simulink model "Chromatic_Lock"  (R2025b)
settings: Solver=FixedStepDiscrete  StartTime=0.0  StopTime=inf  FixedStep=0.01  RelTol=1e-3  EnableMultiTasking=on
libraries: arduinolib x3
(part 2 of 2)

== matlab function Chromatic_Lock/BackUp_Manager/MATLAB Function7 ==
function [RGB, L1, L2, L3, L4, Tone_Event] = ...
    Game_Manager(R_idx, G_idx, B_idx, Match_Btn, Select_Btn, Difficulty_Input, Reset_Btn)
%#codegen

%% ================= DATA TYPES =================
R_idx = uint8(R_idx);
G_idx = uint8(G_idx);
B_idx = uint8(B_idx);
Difficulty_Input = uint8(Difficulty_Input);

% Clamp encoder indices to valid palette range
R_idx = max(uint8(1), min(uint8(6), R_idx));
G_idx = max(uint8(1), min(uint8(6), G_idx));
B_idx = max(uint8(1), min(uint8(6), B_idx));

% Clamp difficulty
Difficulty_Input = max(uint8(1), min(uint8(3), Difficulty_Input));

%% ============ PERSISTENT VARIABLES ============
persistent state puzzle_count puzzle_limit ...
    R_tgt G_tgt B_tgt ...
    R_hints G_hints B_hints

if isempty(state)
    state = uint8(0);  % welcome screen        % 0=Select Difficulty, 1=Play, 2=Complete
    puzzle_count = uint8(1);
    puzzle_limit = uint8(0);

    % --- Targets as numeric arrays (6 puzzles) ---
    R_tgt = zeros(6,1,'uint8');
    G_tgt = zeros(6,1,'uint8');
    B_tgt = zeros(6,1,'uint8');

    % --- Hints as cell arrays (6 puzzles x 3 difficulty levels) ---
    R_hints = cell(6,3);
    G_hints = cell(6,3);
    B_hints = cell(6,3);

    % ==================== PUZZLES ====================
    % PUZZLE 1
    R_tgt(1) = 2; R_hints{1,1} = 'Rot: Tomatenrot      '; R_hints{1,2} = 'Rot: Ziegelrot       '; R_hints{1,3} = 'Rot: Scharlach       ';
    G_tgt(1) = 1; G_hints{1,1} = 'Gruen: Apfelgruen    '; G_hints{1,2} = 'Gruen: Fruehlingsgruen'; G_hints{1,3} = 'Gruen: Moosgruen      ';
    B_tgt(1) = 3; B_hints{1,1} = 'Blau: Azurblau       '; B_hints{1,2} = 'Blau: EU-Blau        '; B_hints{1,3} = 'Blau: Koenigsblau     ';

    % PUZZLE 2
    R_tgt(2) = 4; R_hints{2,1} = 'Rot: Kirschrot       '; R_hints{2,2} = 'Rot: Rubinrot        '; R_hints{2,3} = 'Rot: Purpur          ';
    G_tgt(2) = 3; G_hints{2,1} = 'Gruen: Hoffnungsgruen'; G_hints{2,2} = 'Gruen: Smaragd       '; G_hints{2,3} = 'Gruen: Tannengruen    ';
    B_tgt(2) = 5; B_hints{2,1} = 'Blau: Marineblau     '; B_hints{2,2} = 'Blau: Tiefsee        '; B_hints{2,3} = 'Blau: Mitternacht    ';

    % PUZZLE 3
    R_tgt(3) = 6; R_hints{3,1} = 'Rot: Feuerrot        '; R_hints{3,2} = 'Rot: Glutrot         '; R_hints{3,3} = 'Rot: Vulkanrot       ';
    G_tgt(3) = 1; G_hints{3,1} = 'Gruen: Apfelgruen    '; G_hints{3,2} = 'Gruen: Limette       '; G_hints{3,3} = 'Gruen: Farn          ';
    B_tgt(3) = 3; B_hints{3,1} = 'Blau: Heraldik       '; B_hints{3,2} = 'Blau: Stahlblau      '; B_hints{3,3} = 'Blau: Polarblau      ';

    % PUZZLE 4
    R_tgt(4) = 3; R_hints{4,1} = 'Rot: Ziegelrot       '; R_hints{4,2} = 'Rot: Terrakotta      '; R_hints{4,3} = 'Rot: Ockerrot        ';
    G_tgt(4) = 4; G_hints{4,1} = 'Gruen: Limettengruen '; G_hints{4,2} = 'Gruen: Chartreuse    '; G_hints{4,3} = 'Gruen: Neon          ';
    B_tgt(4) = 2; B_hints{4,1} = 'Blau: Mittelmeer     '; B_hints{4,2} = 'Blau: Kuestenblau    '; B_hints{4,3} = 'Blau: Horizont       ';

    % PUZZLE 5
    R_tgt(5) = 5; R_hints{5,1} = 'Rot: Rosenrot        '; R_hints{5,2} = 'Rot: Altrosa         '; R_hints{5,3} = 'Rot: Pastellrot      ';
    G_tgt(5) = 6; G_hints{5,1} = 'Gruen: Dschungelgruen'; G_hints{5,2} = 'Gruen: Tropengruen   '; G_hints{5,3} = 'Gruen: Mangroven     ';
    B_tgt(5) = 1; B_hints{5,1} = 'Blau: Eisblau        '; B_hints{5,2} = 'Blau: EU-Blau        '; B_hints{5,3} = 'Blau: Stahlblau      ';

    % PUZZLE 6
    R_tgt(6) = 1; R_hints{6,1} = 'Rot: Tomatenrot      '; R_hints{6,2} = 'Rot: Bordeaux        '; R_hints{6,3} = 'Rot: Burgunder       ';
    G_tgt(6) = 2; G_hints{6,1} = 'Gruen: Irischgruen   '; G_hints{6,2} = 'Gruen: Moosgruen     '; G_hints{6,3} = 'Gruen: Waldgruen     ';
    B_tgt(6) = 5; B_hints{6,1} = 'Blau: Marineblau     '; B_hints{6,2} = 'Blau: Tiefsee        '; B_hints{6,3} = 'Blau: Nachtblau      ';
end

%% ================= RESET ======================
if Reset_Btn
    state = uint8(0);   % welcome screen
    puzzle_count = uint8(1);
    puzzle_limit = uint8(0);
end

%% ================= DEFAULT OUTPUTS ============
RGB = [0.2 0.2 0.2];
Tone_Event = uint8(0);

L1 = uint8('                    ');
L2 = uint8('                    ');
L3 = uint8('                    ');
L4 = uint8('                    ');

palette = [1.0 0.8 0.6 0.4 0.2 0.1];

%% ================= FSM ========================
switch state

    % ========== STATE 0: WELCOME SCREEN ==========
    case 0
        L1 = uint8('   Chromatic Lock   ');
        L2 = uint8('       Bereit       ');
        L3 = uint8('                    ');
        L4 = uint8('Druecke zum Starten ');

        if Select_Btn
            state = uint8(1);
        end

    % ========== STATE 1: SELECT DIFFICULTY ==========
    case 1
        L1 = uint8('-- SCHWIERIGKEIT -- ');

        % --- Visual feedback for selection ---
        if Difficulty_Input == 1
            L2 = uint8('> 1 LEICHT          ');
            L3 = uint8('  2 MITTEL          ');
            L4 = uint8('  3 SCHWER          ');
        elseif Difficulty_Input == 2
            L2 = uint8('  1 LEICHT          ');
            L3 = uint8('> 2 MITTEL          ');
            L4 = uint8('  3 SCHWER          ');
        elseif Difficulty_Input == 3
            L2 = uint8('  1 LEICHT          ');
            L3 = uint8('  2 MITTEL          ');
            L4 = uint8('> 3 SCHWER          ');
        end

        if Select_Btn
            if Difficulty_Input == 1
                puzzle_limit = uint8(3);
            elseif Difficulty_Input == 2
                puzzle_limit = uint8(4);
            elseif Difficulty_Input == 3
                puzzle_limit = uint8(6);
            else
                puzzle_limit = uint8(0);
            end

            if puzzle_limit > 0
                Tone_Event = uint8(1);
                puzzle_count = uint8(1);
                state = uint8(2);
            end
        end

    % ========== STATE 2: PLAY GAME ==========
    case 2
        tgtR = R_tgt(puzzle_count);
        tgtG = G_tgt(puzzle_count);
        tgtB = B_tgt(puzzle_count);

        RGB = [palette(R_idx), palette(G_idx), palette(B_idx)];

        diffIdx = Difficulty_Input;

        L1 = uint8('Mische RGB nach Hint');

        r_hint = char(R_hints{puzzle_count, diffIdx});
        g_hint = char(G_hints{puzzle_count, diffIdx});
        b_hint = char(B_hints{puzzle_count, diffIdx});

        if length(r_hint) < 20, r_hint = [r_hint, repmat(' ',1,20-length(r_hint))]; end
        if length(g_hint) < 20, g_hint = [g_hint, repmat(' ',1,20-length(g_hint))]; end
        if length(b_hint) < 20, b_hint = [b_hint, repmat(' ',1,20-length(b_hint))]; end

        L2 = zeros(1,20,'uint8');
        L3 = zeros(1,20,'uint8');
        L4 = zeros(1,20,'uint8');
        for i = 1:20
            L2(i) = uint8(r_hint(i));
            L3(i) = uint8(g_hint(i));
            L4(i) = uint8(b_hint(i));
        end

        if Match_Btn
            if R_idx == tgtR && G_idx == tgtG && B_idx == tgtB
                Tone_Event = uint8(2);
                if puzzle_count < puzzle_limit
                    puzzle_count = puzzle_count + 1;
                else
                    state = uint8(3);
                end
            else
                Tone_Event = uint8(3);
            end
        end

    % ========== STATE 3: GAME COMPLETE ==========
    case 3
        RGB = [0 1 0];
        Tone_Event = uint8(2);

        L1 = uint8('***   GLUECKWUNSCH  ');
        L2 = uint8('Alle Raetsel geloest');
        L3 = uint8('GEHEIMCODE:     4729');
        L4 = uint8('Reset fuer Neustart ');
end
end

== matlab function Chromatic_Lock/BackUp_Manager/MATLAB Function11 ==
function [RGB, L1, L2, L3, L4, Buzzer] = ...
    Game_Manager(R_idx, G_idx, B_idx, Match_Btn, Select_Btn, Difficulty_Input, Reset_Btn)
%#codegen

%% ================= DATA TYPES =================
R_idx = uint8(R_idx);
G_idx = uint8(G_idx);
B_idx = uint8(B_idx);
Difficulty_Input = uint8(Difficulty_Input);

%% ============ PERSISTENT VARIABLES ============
persistent state puzzle_count puzzle_limit targets

if isempty(state)
    state = uint8(0);        % 0=Select Difficulty, 1=Play, 2=Complete
    puzzle_count = uint8(1);
    puzzle_limit = uint8(0);

    targets = uint8([ ...
        2 1 3;
        4 3 5;
        6 1 3;
        3 4 2;
        5 6 1;
        1 2 5 ]);
end

%% ================= RESET ======================
if Reset_Btn
    state = uint8(0);
    puzzle_count = uint8(1);
    puzzle_limit = uint8(0);
end

%% ================= DEFAULT OUTPUTS ============
RGB = [0.2 0.2 0.2];
Buzzer = false;

L1 = uint8('                    ');
L2 = uint8('                    ');
L3 = uint8('                    ');
L4 = uint8('                    ');

palette = [1.0 0.8 0.6 0.4 0.2 0.1];

%% ================= FSM ========================
switch state

    % ========== STATE 0: SELECT DIFFICULTY ==========
    case 0
        L1 = uint8('--- SELECT LEVEL ---');
        L2 = uint8('1 Easy 2 Med 3 Hard ');
        L3 = uint8('Choose & Press SEL  ');
        L4 = uint8('                    ');

        if Select_Btn
            if Difficulty_Input == 1
                puzzle_limit = uint8(3);
            elseif Difficulty_Input == 2
                puzzle_limit = uint8(4);
            elseif Difficulty_Input == 3
                puzzle_limit = uint8(6);
            else
                puzzle_limit = uint8(0); % invalid selection
            end

            if puzzle_limit > 0
                puzzle_count = uint8(1);
                state = uint8(1);
            end
        end

    % ========== STATE 1: PLAY GAME ==========
    case 1
        tgt = targets(puzzle_count, :);

        % Live RGB mixing
        RGB = [ palette(R_idx), ...
                palette(G_idx), ...
                palette(B_idx) ];

        % LCD Hint Layout (AS REQUESTED)
        L1 = uint8('--- HINT SECTION ---');
        L2 = redHint(tgt(1));
        L3 = greenHint(tgt(2));
        L4 = blueHint(tgt(3));

        % Match check (ONE PUZZLE AT A TIME)
        if Match_Btn && ...
           R_idx == tgt(1) && ...
           G_idx == tgt(2) && ...
           B_idx == tgt(3)

            if puzzle_count < puzzle_limit
                puzzle_count = puzzle_count + 1;
            else
                state = uint8(2);
            end
        end

    % ========== STATE 2: GAME COMPLETE ==========
    case 2
        RGB = [0 1 0];
        Buzzer = true;

        L1 = uint8('*** CONGRATULATIONS ');
        L2 = uint8('ALL PUZZLES SOLVED  ');
        L3 = uint8('SECRET CODE:        ');
        L4 = uint8('4729                ');
end
end

%% ============ HINT FUNCTIONS ==================
function t = redHint(i)
h = uint8(['Red: Tomato         ';
           'Red: Bordeaux       ';
           'Red: Brick          ';
           'Red: Cherry         ';
           'Red: Rose           ';
           'Red: Fire           ']);
t = h(i,:);
end

function t = greenHint(i)
h = uint8(['Green: Apple        ';
           'Green: Irish        ';
           'Green: Hope         ';
           'Green: Lime         ';
           'Green: Forest       ';
           'Green: Jungle       ']);
t = h(i,:);
end

function t = blueHint(i)
h = uint8(['Blue: EU Blue       ';
           'Blue: Med Blue      ';
           'Blue: Heraldic      ';
           'Blue: Sky           ';
           'Blue: Navy          ';
           'Blue: Arctic        ']);
t = h(i,:);
end
